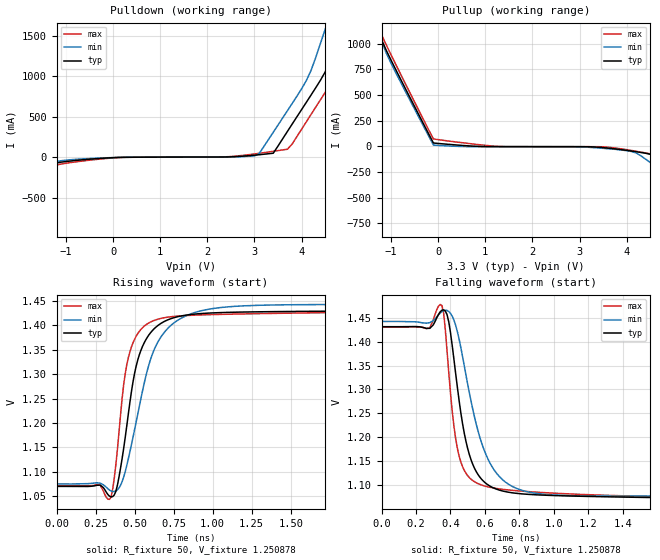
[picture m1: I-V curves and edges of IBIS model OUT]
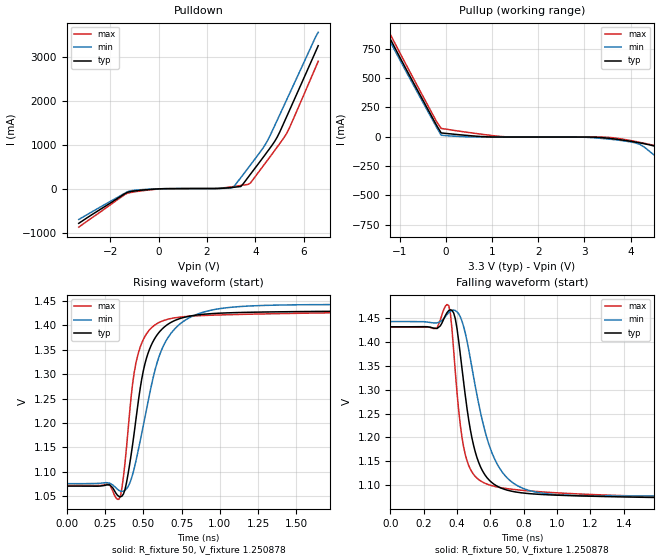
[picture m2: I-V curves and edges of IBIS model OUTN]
|   IBIS File of SG2520VGN C
|   LVDS, Vcc=3.3V, Io=3.5mA, fo<=212.5MHz
[IBIS Ver]   3.2
[File Name]   sg2520vgn_35m_33v.ibs
[File Rev]   1.0
[Date]   Sep. 11, 2020
[Source]
Fairchild Ensigna Lab's Method
[Notes]
Created by Minoru Kozaki
[Disclaimer]
Seiko Epson Corporation makes no warranty with respect to the
information contained herein.
[Copyright]
Copyright(C) 2020, Seiko Epson Corporation. All rights reserved.
|   Component
[Component]   SG2520VGN
[Manufacturer]  Seiko Epson Corporation
[Package]
R_pkg   17.7m   NA   NA
L_pkg   235p   NA   NA
C_pkg   208f   NA   NA
[Pin]   signal_name   model_name   R_pin   L_pin   C_pin
1   OE/ST   NC
2   NC   NC
3   GND   GND
4   OUT   OUT   17.7m   235p   208f
5   OUTN   OUTN   10.4m   129p   221f
6   VCC   POWER
[Diff Pin] inv_pin  vdiff  tdelay_typ
4   5   0   0
| Models and submodels in the file (2): OUT (Output), OUTN (Output)
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|   Model OUT
[Model]   OUT
Model_type   Output
Polarity   Non-Inverting
Vref = 1.25
Vmeas = 1.25
Rref = 50
Cref = 0
C_comp   4.5p   4.5p   4.5p
[Temperature Range]   25   105   -40
[Voltage Range]   3.3   2.97   3.63
[Pullup Reference]   3.3   2.97   3.63
[Pulldown Reference]   0   0   0
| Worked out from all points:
|   slope of the pulldown table from 0 to 0.495 V, typ, clamps not added: 93.5 ohm
|   slope of the pullup table from 0 to 0.495 V, typ, clamps not added: 26.5 ohm
|   falling waveform, R_fixture 50, V_fixture 1.250878: 20-80 % time 109ps typ, 156ps min, 80.2ps max; typ from 1.43 V to 1.07 V
|   rising waveform, R_fixture 50, V_fixture 1.250878: 20-80 % time 126ps typ, 179ps min, 93.5ps max; typ from 1.07 V to 1.43 V
[Pullup]
-3.3V     4.634A     4.475A     4.808A
-1.3V     1.175A     1.177A     1.202A
-1.1V     934.7mA    908.2mA    987.6mA
-1V       840.2mA    810.3mA    892.6mA
-100mV    31.91mA    11.67mA    71.37mA
1.3V      -3.437mA   -3.592mA   -1.697mA
3.6V      -17.53mA   -23.59mA   -8.955mA
4.2V      -53.13mA   -64.93mA   -48.42mA
4.5V      -77.62mA   -157.9mA   -73.53mA
4.6V      -97.25mA   -190.7mA   -82.62mA
5V        -243.6mA   -321.1mA   -145.1mA
6.6V      -825.2mA   -837.5mA   -802.7mA
[Pulldown]
-3.3V     -816.1mA   -723.1mA   -918.3mA
-1.2V     -68mA      -51.8mA    -92.85mA
100mV     -774.1uA   -238.6uA   -2.802mA
3V        27.56mA    17.93mA    42.54mA
3.4V      51.43mA    310.9mA    75.26mA
3.8V      410.6mA    665.2mA    164.4mA
4.2V      768.8mA    1.072A     529.1mA
4.5V      1.053A     1.58A      801.5mA
4.8V      1.538A     2.103A     1.078A
4.9V      1.721A     2.278A     1.18A
5.2V      2.272A     2.804A     1.692A
6.6V      4.636A     5.026A     4.227A
[Falling Waveform]
R_fixture = 50
V_fixture = 1.250878
V_fixture_min = 1.258588
V_fixture_max = 1.251410
0s        1.431V     1.442V     1.43V
280ps     1.428V     1.44V      1.429V
350ps     1.466V     1.463V     1.475V
390ps     1.441V     1.463V     1.336V
420ps     1.363V     1.445V     1.223V
460ps     1.252V     1.388V     1.149V
550ps     1.128V     1.227V     1.105V
700ps     1.088V     1.112V     1.092V
1.05ns    1.078V     1.079V     1.082V
4ns       1.07V      1.076V     1.072V
[Rising Waveform]
R_fixture = 50
V_fixture = 1.250878
V_fixture_min = 1.258588
V_fixture_max = 1.251410
0s        1.07V      1.075V     1.072V
340ps     1.05V      1.063V     1.044V
390ps     1.073V     1.063V     1.146V
430ps     1.148V     1.089V     1.279V
470ps     1.243V     1.141V     1.346V
540ps     1.349V     1.25V      1.392V
650ps     1.4V       1.367V     1.413V
820ps     1.421V     1.418V     1.42V
1.15ns    1.427V     1.439V     1.423V
4ns       1.431V     1.442V     1.43V
[Ramp]
R_load = 50
dV/dt_r   0.21657/126.21p   0.21944/177.94p   0.21571/94.24p
dV/dt_f   0.21657/109.31p   0.21944/155.24p   0.21571/80.05p
|   Model OUTN
[Model]   OUTN
Model_type   Output
Polarity   Inverting
Vref = 1.25
Vmeas = 1.25
Rref = 50
Cref = 0
C_comp   4.5p   4.5p   4.5p
[Temperature Range]   25   105   -40
[Voltage Range]   3.3   2.97   3.63
[Pullup Reference]   3.3   2.97   3.63
[Pulldown Reference]   0   0   0
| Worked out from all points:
|   slope of the pulldown table from 0 to 0.495 V, typ, clamps not added: 93.8 ohm
|   slope of the pullup table from 0 to 0.495 V, typ, clamps not added: 26.7 ohm
|   falling waveform, R_fixture 50, V_fixture 1.250878: 20-80 % time 111ps typ, 156ps min, 82.6ps max; typ from 1.43 V to 1.07 V
|   rising waveform, R_fixture 50, V_fixture 1.250878: 20-80 % time 127ps typ, 179ps min, 94.9ps max; typ from 1.07 V to 1.43 V
[Pullup]
-3.3V     3.26A      3.195A     3.331A
-1.4V     985.5mA    966.6mA    1.027A
-1.3V     907.8mA    884.7mA    949.2mA
-1.2V     831.8mA    808.1mA    872.3mA
-200mV    96.81mA    80.51mA    128mA
-100mV    31.65mA    11.63mA    70.25mA
1.3V      -3.437mA   -3.592mA   -1.705mA
3.4V      -9.276mA   -16.29mA   -4.073mA
4.1V      -46.41mA   -53.19mA   -40.86mA
4.5V      -79.32mA   -154.4mA   -74.26mA
5V        -234.9mA   -309.3mA   -138.9mA
6.6V      -799.1mA   -817.9mA   -761mA
[Pulldown]
-3.3V     -789.4mA   -702mA     -877.2mA
-1.3V     -85.14mA   -73.25mA   -105.8mA
100mV     -773.4uA   -238.3uA   -2.8mA
2.3V      4.743mA    4.465mA    5.439mA
3.1V      32.91mA    37.3mA     49.85mA
3.4V      51.01mA    253.7mA    74.38mA
3.8V      333.4mA    543.1mA    131.8mA
4.5V      848.4mA    1.094A     649.2mA
4.9V      1.175A     1.559A     949mA
5.2V      1.528A     1.916A     1.179A
5.4V      1.775A     2.155A     1.378A
6.6V      3.266A     3.571A     2.909A
[Falling Waveform]
R_fixture = 50
V_fixture = 1.250878
V_fixture_min = 1.258588
V_fixture_max = 1.251410
0s        1.431V     1.442V     1.43V
280ps     1.427V     1.439V     1.429V
340ps     1.461V     1.457V     1.478V
370ps     1.465V     1.465V     1.425V
420ps     1.372V     1.451V     1.225V
470ps     1.237V     1.383V     1.142V
580ps     1.116V     1.198V     1.103V
710ps     1.089V     1.113V     1.093V
1.1ns     1.078V     1.079V     1.083V
4ns       1.071V     1.076V     1.072V
[Rising Waveform]
R_fixture = 50
V_fixture = 1.250878
V_fixture_min = 1.258588
V_fixture_max = 1.251410
0s        1.071V     1.076V     1.072V
340ps     1.05V      1.062V     1.044V
390ps     1.078V     1.065V     1.15V
430ps     1.156V     1.095V     1.281V
460ps     1.228V     1.134V     1.334V
530ps     1.342V     1.243V     1.387V
650ps     1.4V       1.369V     1.412V
820ps     1.42V      1.419V     1.419V
1.15ns    1.426V     1.439V     1.422V
4ns       1.431V     1.442V     1.43V
[Ramp]
R_load = 50
dV/dt_r   0.21553/126.45p   0.21840/177.06p   0.21468/95.01p
dV/dt_f   0.21553/110.64p   0.21840/155.40p   0.21468/82.26p
